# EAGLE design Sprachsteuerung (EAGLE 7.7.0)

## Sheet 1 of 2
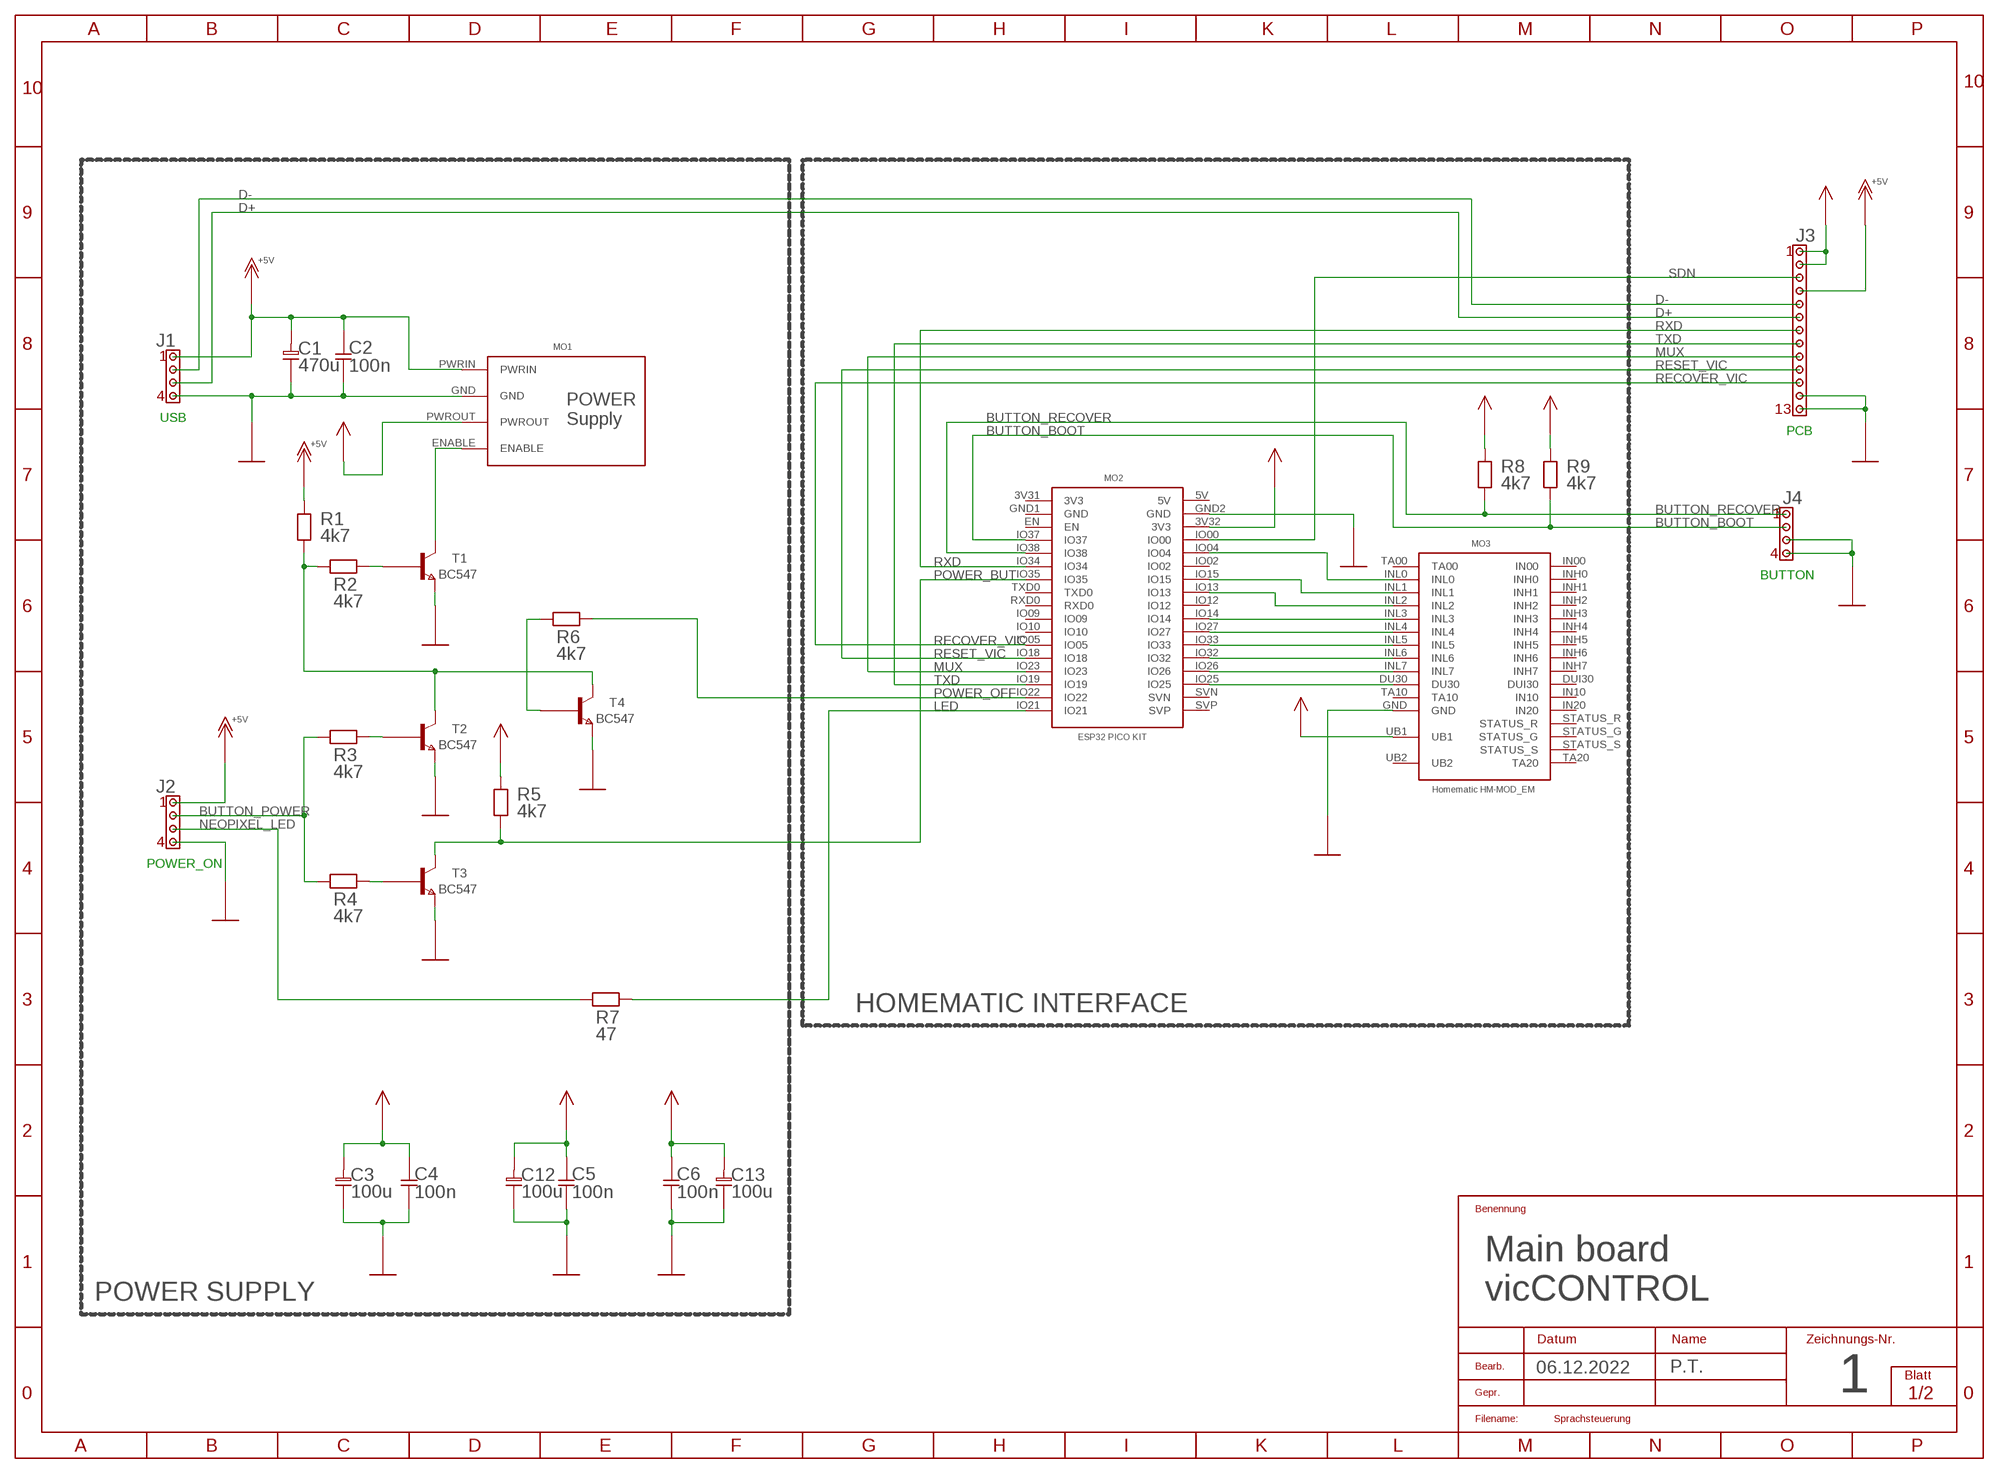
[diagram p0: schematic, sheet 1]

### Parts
C1  470u  ELK02ST  [ELKOS02B]
C2  100n  CAP02  [CAP02B]
C3  100u  ELK02ST  [ELKOS02B]
C4  100n  CAP02  [CAP02B]
C5  100n  CAP02  [CAP02B]
C6  100n  CAP02  [CAP02B]
C12  100u  ELK02ST  [ELKOS02B]
C13  100u  ELK02ST  [ELKOS02B]
J1  POWER_ON  CON04X1  [CON04X1]
J2  POWER_ON  CON04X1  [CON04X1]
J3  PCB  CON13X1  [CON13X1]
J4  BUTTON  CON04X1  [CON04X1]
MO1  POWER_SUPPLY  [POWER_SUPPLY]
MO2  ESP32-PICO-KIT  [ESP32-PICO-KIT]
MO3  HM_MOD_EM  [HM_MOD_EM]
R1  4k7  RES01  [RES01B]
R2  4k7  RES01  [RES01B]
R3  4k7  RES01  [RES01B]
R4  4k7  RES04  [RES04B]
R5  4k7  RES02  [RES02B]
R6  4k7  RES04  [RES04B]
R7  47  RES04  [RES04B]
R8  4k7  RES02  [RES02B]
R9  4k7  RES04  [RES04B]
T1  BC547  [TO92A]
T2  BC547  [TO92A]
T3  BC547  [TO92A]
T4  BC547  [TO92A]

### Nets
+5V: C1.P C2.2 J1.1 J2.1 J3.4 MO1.PWRIN R1.2
BUTTON_BOOT: J4.2 MO2.IO37 R9.1
BUTTON_POWER: J2.2 R3.1 R4.1
BUTTON_RECOVER: J4.1 MO2.IO38 R8.1
D+: J1.3 J3.6
D-: J1.2 J3.5
GND: C1.N C2.1 C3.N C4.1 C5.1 C6.1 C12.N C13.N J1.4 J2.4 J3.12 J3.13 J4.3 J4.4 MO1.GND MO2.GND2(GND) MO3.GND T1.3(E) T2.3(E) T3.3(E) T4.3(E)
LED: MO2.IO21 R7.2
MUX: J3.9 MO2.IO23
N$1: MO1.ENABLE T1.1(C)
N$2: R2.2 T1.2(B)
N$3: MO2.IO14 MO3.INL3
N$4: R1.1 R2.1 T2.1(C) T4.1(C)
N$5: MO2.IO04 MO3.INL0
N$10: R3.2 T2.2(B)
N$19: R4.2 T3.2(B)
N$21: MO2.IO15 MO3.INL1
N$22: R6.1 T4.2(B)
N$23: MO2.IO13 MO3.INL2
N$25: MO2.IO27 MO3.INL4
N$26: MO2.IO33 MO3.INL5
N$27: MO2.IO32 MO3.INL6
N$28: MO2.IO26 MO3.INL7
N$29: MO2.IO25 MO3.DU30
NEOPIXEL_LED: J2.3 R7.1
POWER_BUT: MO2.IO35 R5.1 T3.1(C)
POWER_OFF: MO2.IO22 R6.2
RECOVER_VIC: J3.11 MO2.IO05
RESET_VIC: J3.10 MO2.IO18
RXD: J3.7 MO2.IO34
SDN: J3.3 MO2.IO00
TXD: J3.8 MO2.IO19
VCC: C3.P C4.2 C5.2 C6.2 C12.P C13.P J3.1 J3.2 MO1.PWROUT MO2.3V32(3V3) MO3.UB1 R5.2 R8.2 R9.2
Unconnected: MO2.EN MO2.IO02 MO2.IO09 MO2.IO10 MO2.IO12 MO2.RXD0 MO2.SVN MO2.SVP MO2.TXD0 MO3.DUI30 MO3.IN00 MO3.IN10 MO3.IN20 MO3.INH0 MO3.INH1 MO3.INH2 MO3.INH3 MO3.INH4 MO3.INH5 MO3.INH6 MO3.INH7 MO3.STATUS_G MO3.STATUS_R MO3.STATUS_S MO3.TA00 MO3.TA10 MO3.TA20

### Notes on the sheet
- USB
- PCB
- BUTTON
- POWER_ON
- HOMEMATIC INTERFACE
- Main board
- POWER SUPPLY | vicCONTROL
- 06.12.2022 | P.T.
- 1

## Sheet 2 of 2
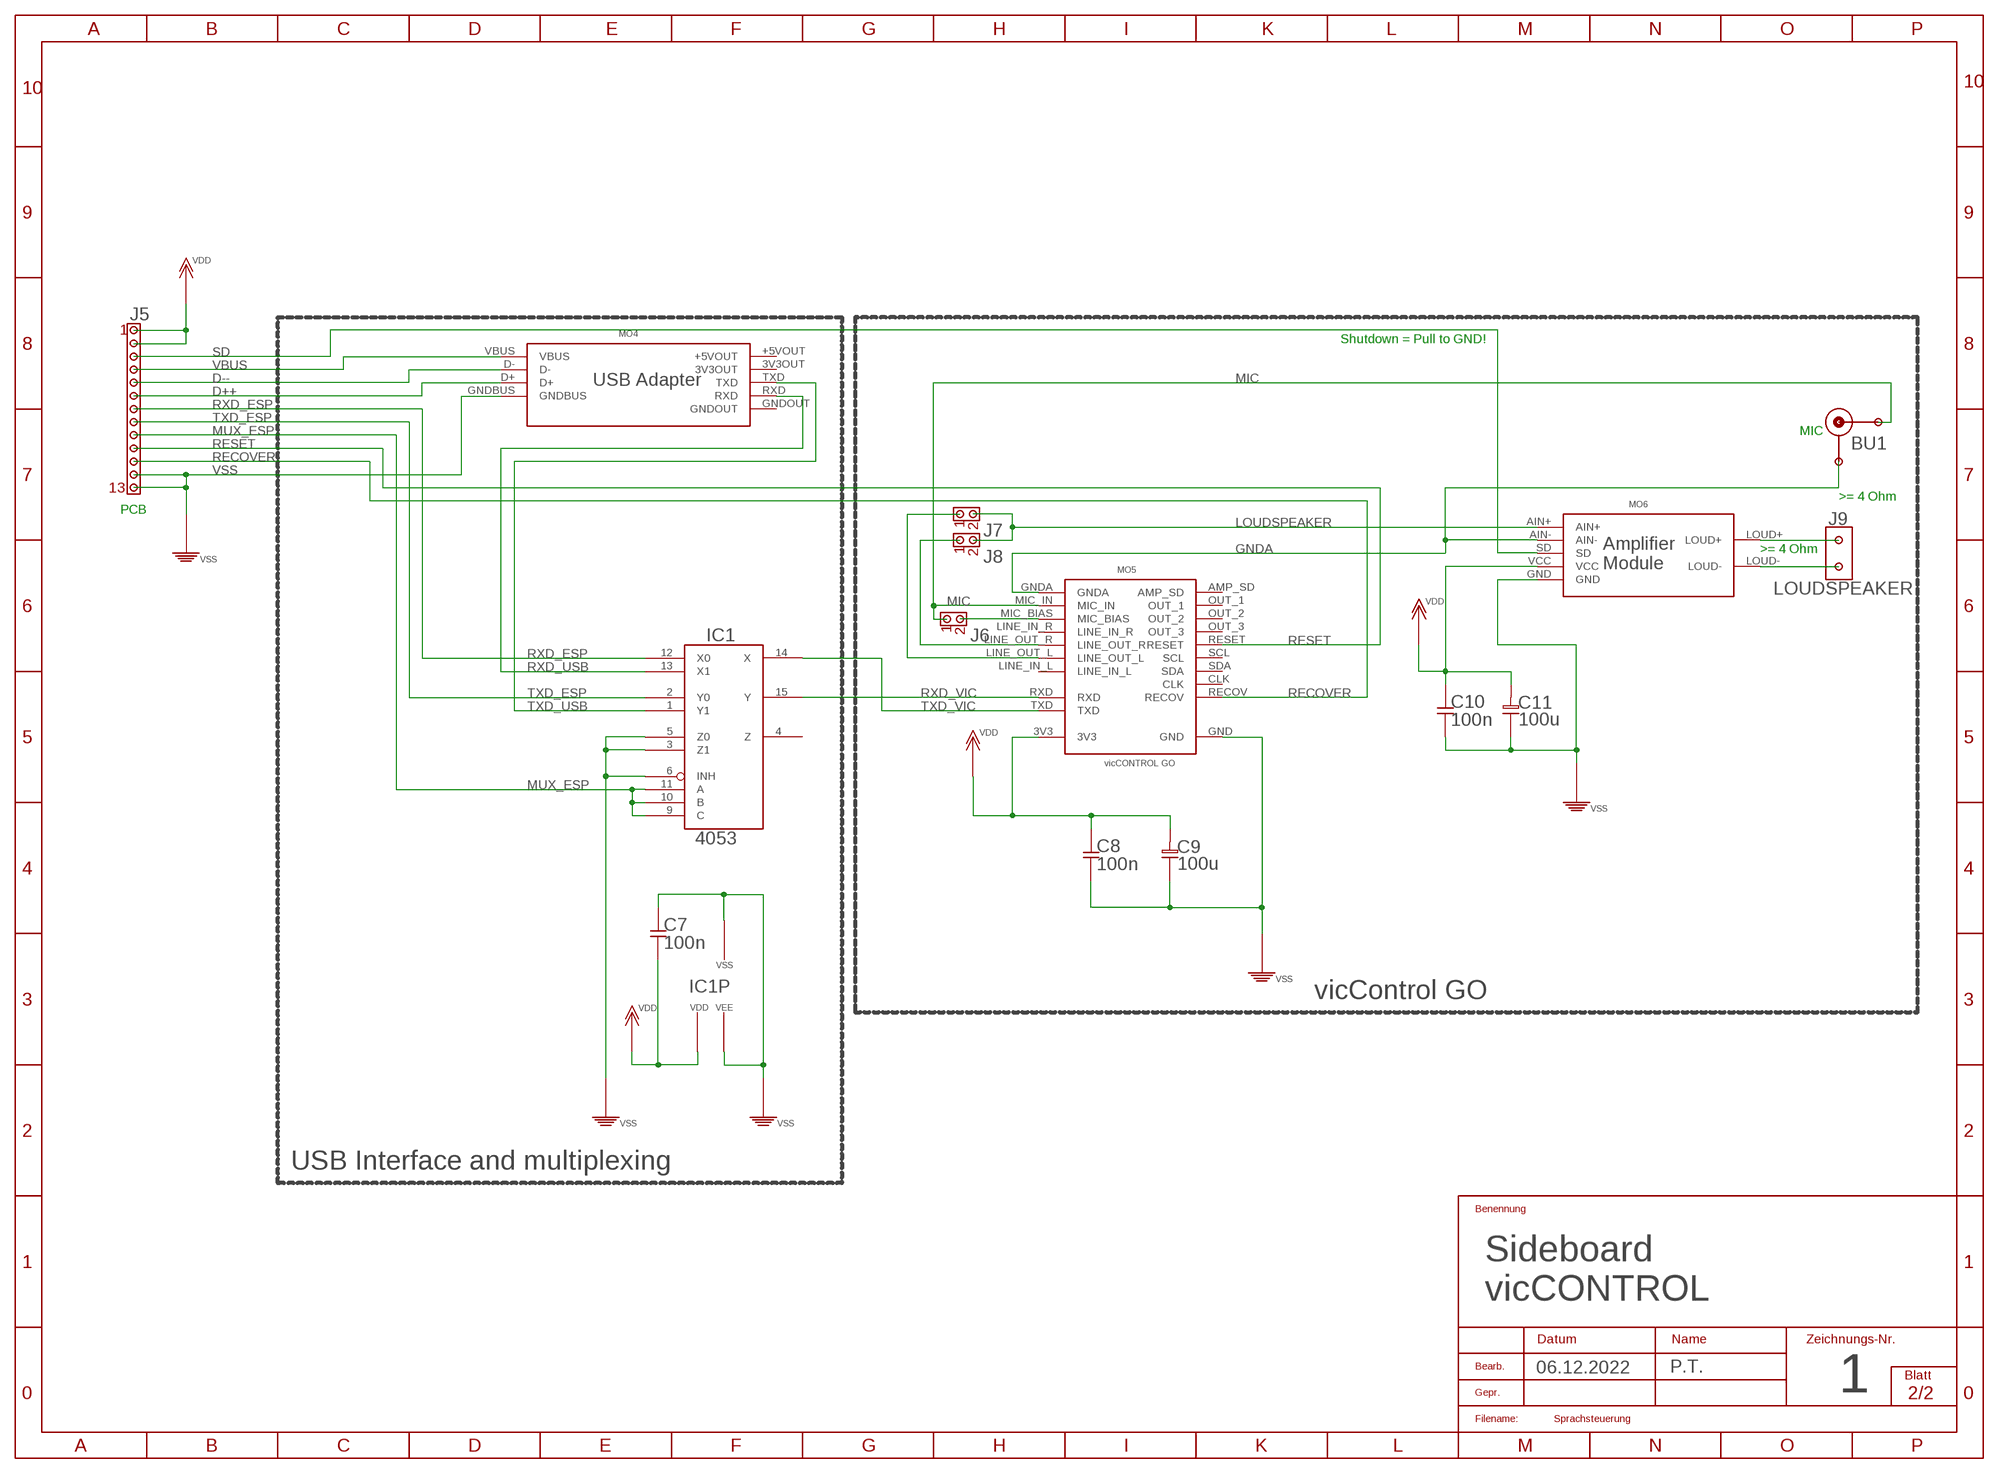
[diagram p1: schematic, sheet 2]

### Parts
BU1  MIC  KLINKE3M  [KLINKE3M]
C7  100n  CAP02  [CAP02B]
C8  100n  CAP02  [CAP02B]
C9  100u  ELK02ST  [ELKOS02B]
C10  100n  CAP02  [CAP02B]
C11  100u  ELK02ST  [ELKOS02B]
IC1  4053  [DIL16]
J5  PCB  CON13X1  [CON13X1]
J6  MIC  CON02X1  [CON02X1]
J7  LINE_L  CON02X1  [CON02X1]
J8  LINE_R  CON02X1  [CON02X1]
J9  LOUDSPEAKER  POWER2X1  [POWER2X1]
MO4  USB-ADAPTER  [USB-ADAPTER]
MO5  VIC-CONTROL-GO  [VIC-CONTROL-GO]
MO6  AMPLIFIER  [AMPLIFIER]

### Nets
D++: J5.6 MO4.D+
D--: J5.5 MO4.D-
GNDA: BU1.GND MO5.GNDA MO6.AIN-
LOUDSPEAKER: J7.2 J8.2 MO6.AIN+
MIC: BU1.IN J6.1 MO5.MIC_IN
MUX_ESP: IC1.9(C) IC1.10(B) IC1.11(A) J5.9
N$6: J6.2 MO5.MIC_BIAS
N$7: J8.1 MO5.LINE_OUT_R
N$8: J7.1 MO5.LINE_OUT_L
N$12: J9.2 MO6.LOUD+
N$13: J9.1 MO6.LOUD-
RECOVER: J5.11 MO5.RECOV
RESET: J5.10 MO5.RESET
RXD_ESP: IC1.12(X0) J5.7
RXD_USB: IC1.13(X1) MO4.RXD
RXD_VIC: IC1.15(Y) MO5.RXD
SD: J5.3 MO6.SD
TXD_ESP: IC1.2(Y0) J5.8
TXD_USB: IC1.1(Y1) MO4.TXD
TXD_VIC: IC1.14(X) MO5.TXD
VBUS: J5.4 MO4.VBUS
VDD: C7.1 C8.2 C9.P C10.2 C11.P IC1.16(VDD) J5.1 J5.2 MO5.3V3 MO6.VCC
VSS: C7.2 C8.1 C9.N C10.1 C11.N IC1.3(Z1) IC1.5(Z0) IC1.6(INH) IC1.7(VEE) IC1.8(VSS) J5.12 J5.13 MO4.GNDBUS MO5.GND MO6.GND
Unconnected: IC1.4(Z) MO5.AMP_SD MO5.CLK MO5.LINE_IN_L MO5.LINE_IN_R MO5.OUT_1 MO5.OUT_2 MO5.OUT_3 MO5.SCL MO5.SDA

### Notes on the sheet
- Shutdown = Pull to GND!
- MIC
- >= 4 Ohm
- PCB
- >= 4 Ohm
- vicControl GO
- USB Interface and multiplexing
- Sideboard
- vicCONTROL
- 06.12.2022 | P.T.
- 1

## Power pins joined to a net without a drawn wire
3V3: MO2.3V31(3V3)
3V3OUT: MO4.3V3OUT
5V: MO2.5V
+5VOUT: MO4.+5VOUT
GND: MO2.GND1(GND)
GNDOUT: MO4.GNDOUT
UB2: MO3.UB2

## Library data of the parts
BU1 = Mechanic:KLINKE3M
C1 C3 C9 C11-C13 = Discrete:ELK02ST
C2 C4-C8 C10 = Discrete:CAP02
IC1 = 40XX:4053
J1 J2 J4 = Connector 1:CON04X1
J3 J5 = Connector 1:CON13X1
J6-J8 = Connector 1:CON02X1
J9 = Connector 2:POWER2X1
MO1 = Giess:POWER_SUPPLY
MO2 = Giess:ESP32-PICO-KIT
MO3 = Giess:HM_MOD_EM
MO4 = Giess:USB-ADAPTER
MO5 = Giess:VIC-CONTROL-GO
MO6 = Giess:AMPLIFIER
R1-R3 = Discrete:RES01
R4 R6 R7 R9 = Discrete:RES04
R5 R8 = Discrete:RES02
T1-T4 = Transistor:BC547

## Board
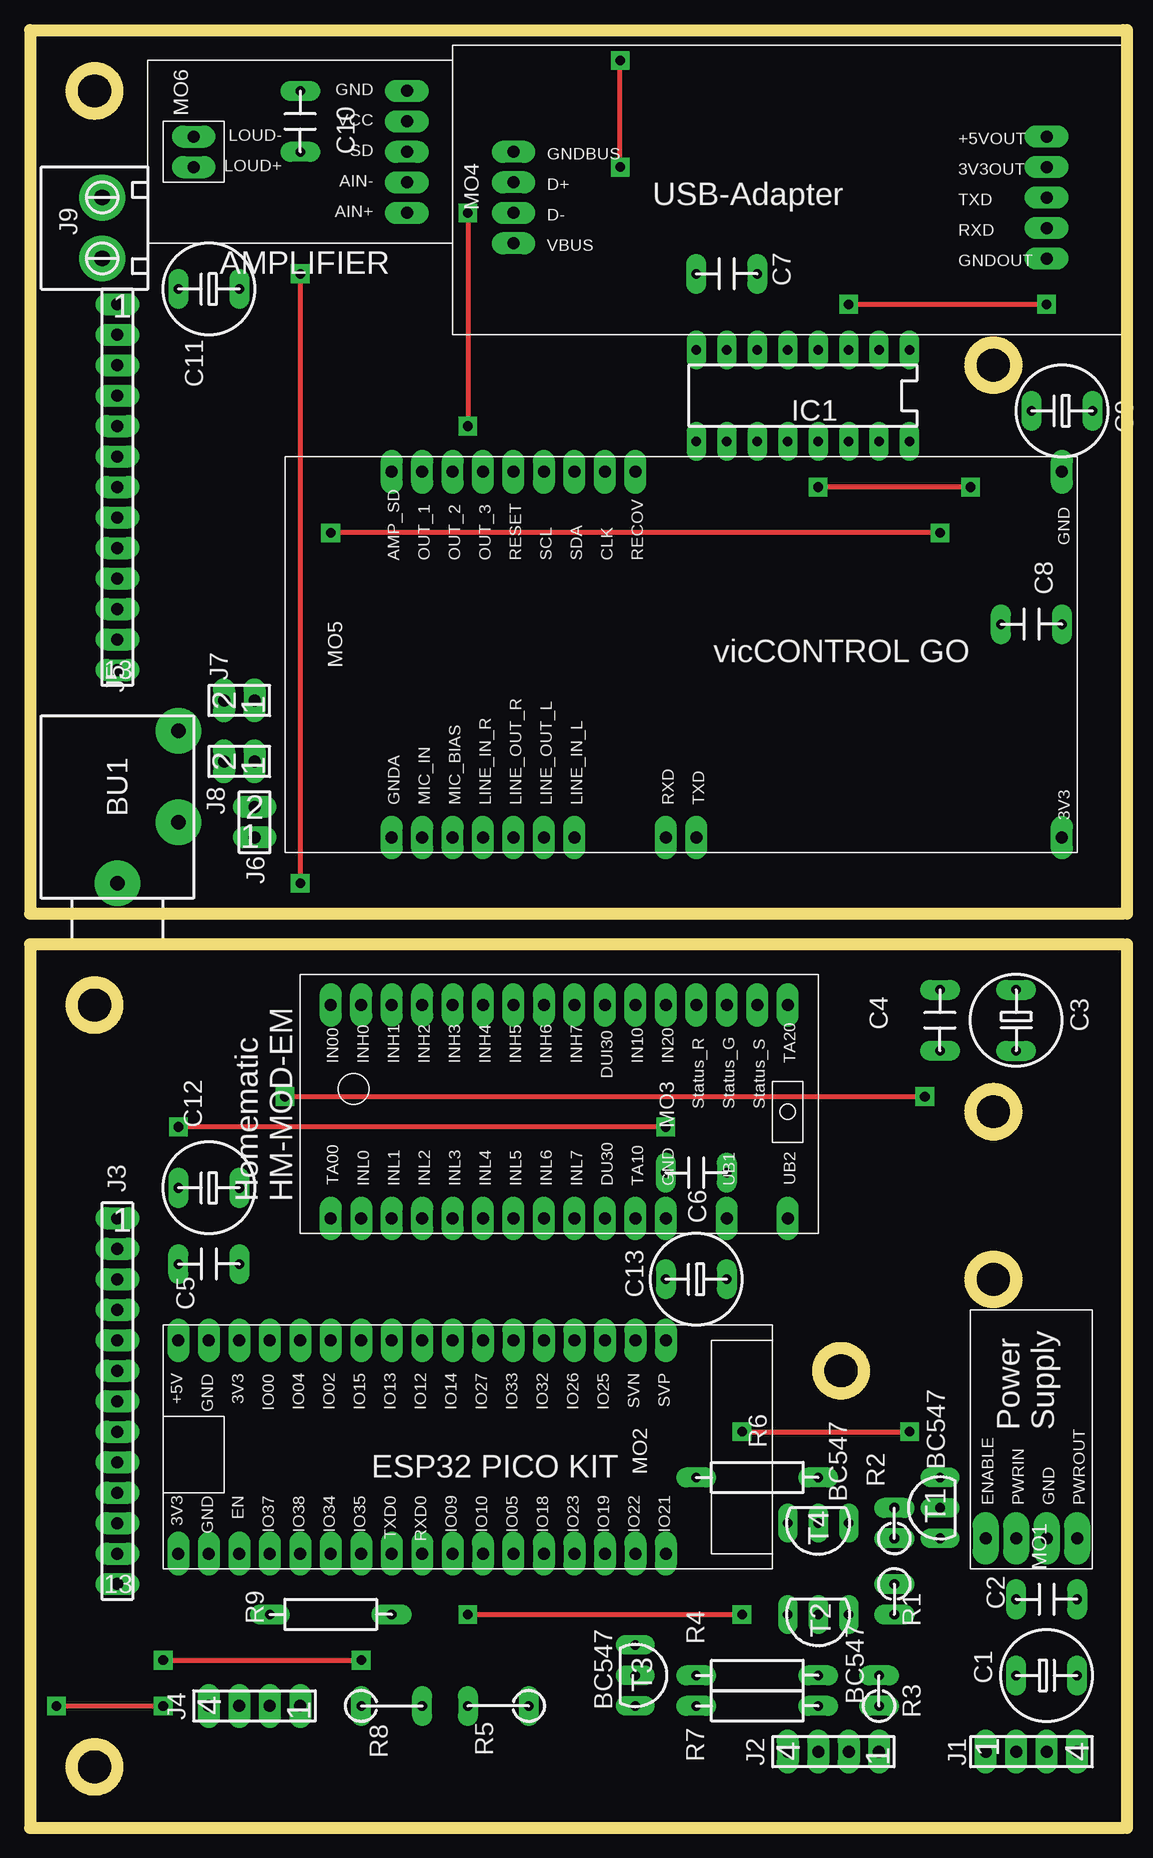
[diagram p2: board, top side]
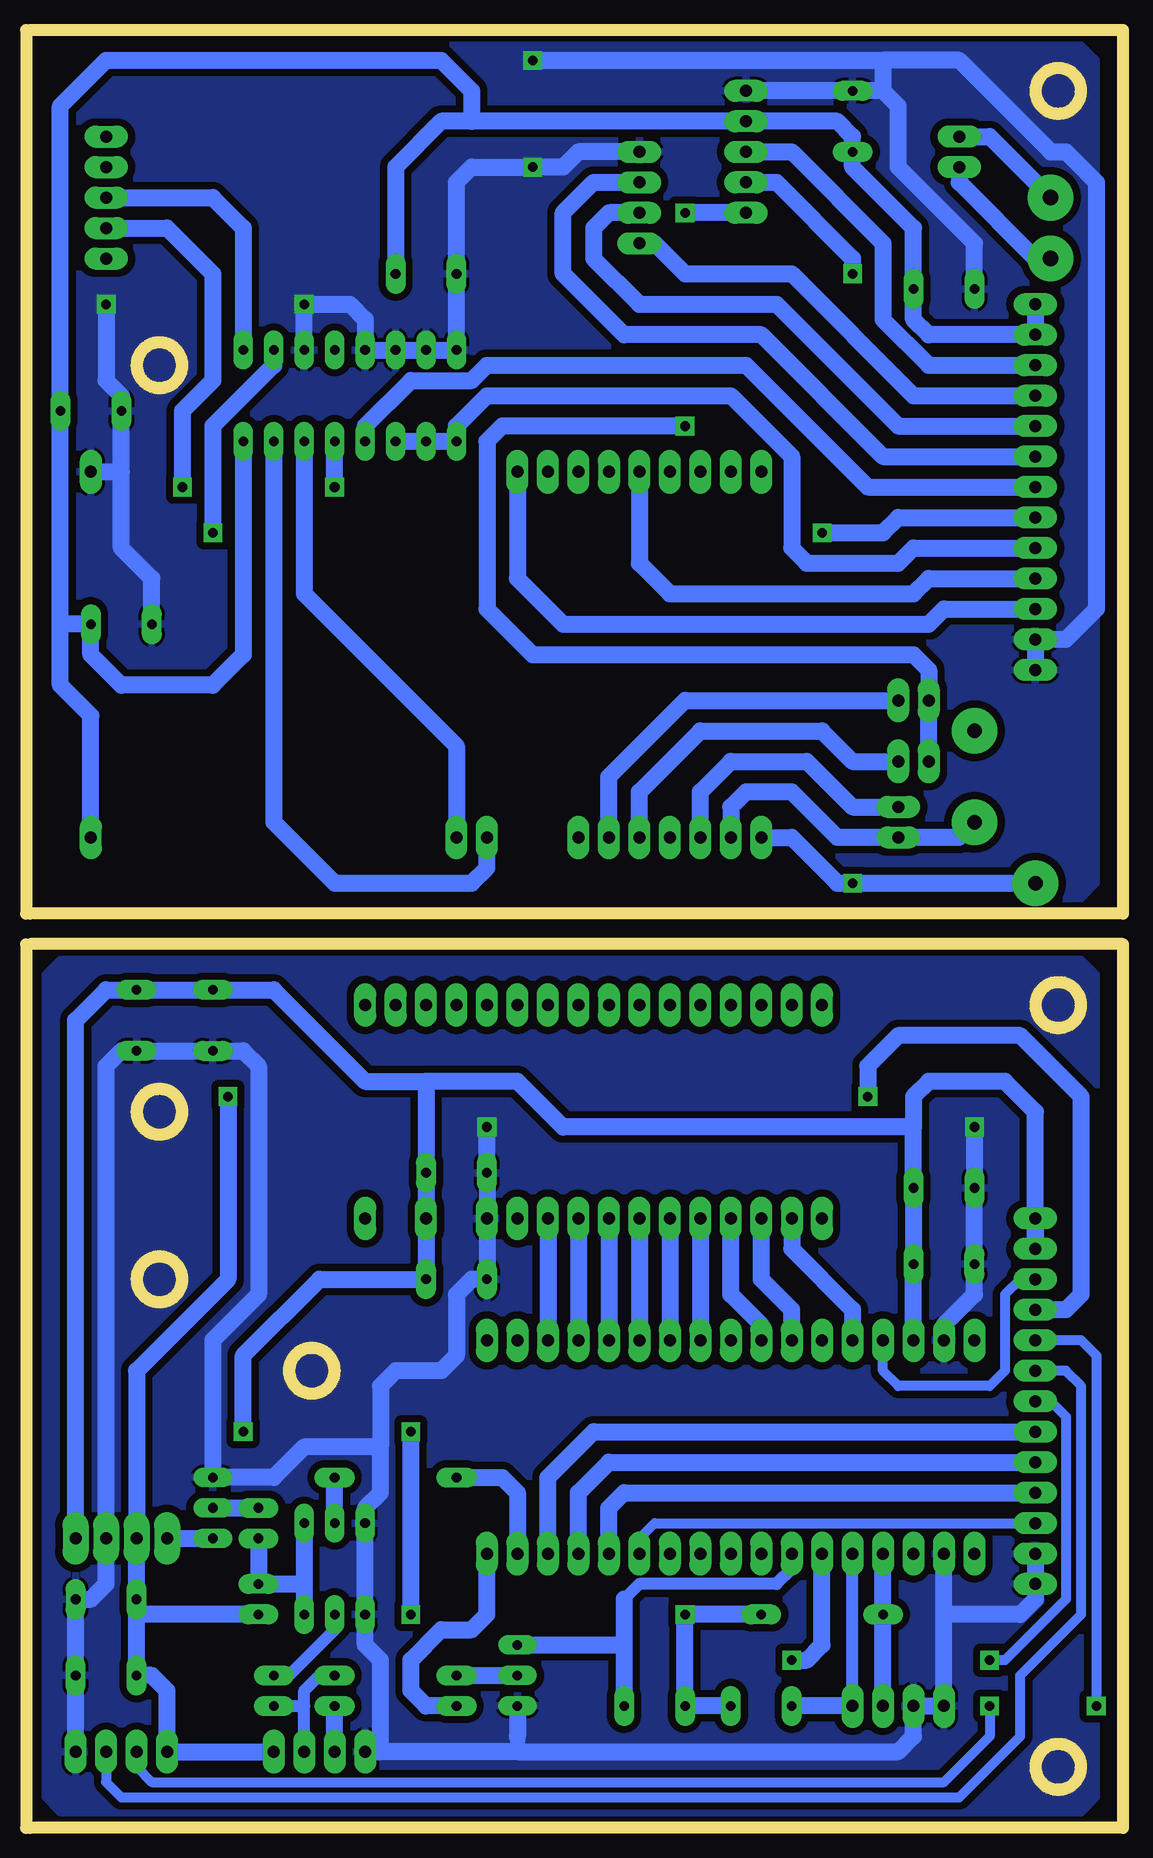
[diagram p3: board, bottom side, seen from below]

Size 91.11 x 149.86 mm. Coordinates in mm from the lower left corner, seen from the top.
Outline: 0,149.84 0,76.2
Outline: 91.11,76.18 0,76.18
Outline: 91.11,76.2 91.11,149.84
Outline: 0,149.86 91.11,149.86
Outline: 91.11,0 91.11,73.64 0,73.64 0,0 91.11,0
Copper layers (1*16): Top 0.035mm / dielectric 1.5mm / Bottom 0.035mm
Design rules "LP_fraesen": minimum track width 16mil, minimum drill 23mil, track to track 8mil, track to pad 8mil, pad to pad 8mil, via to via 8mil, smd to smd 0mil, copper to edge 20mil, drill to drill 8mil, minimum pad ring 16mil, minimum via ring 15mil, stop-mask expansion 4mil, vias tented up to drill 0mil, thermal gap 10mil
Milling: 22 lines

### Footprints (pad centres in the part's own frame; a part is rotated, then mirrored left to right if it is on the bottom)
KLINKE3M = drill 1.2 pad 3.81: GND 0,0; IN 5.08,-5.08; NC 12.7,-5.08
ELKOS02B = drill 0.8 pad 1.676 long: N 5.08,0; P 0,0
CAP02B = drill 0.8 pad 1.676 long: 1 0,0; 2 5.08,0
DIL16 = drill 0.8 pad 1.422 long: 1 0,0; 2 2.54,0; 3 5.08,0; 4 7.62,0; 5 10.16,0; 6 12.7,0; 7 15.24,0; 8 17.78,0; 9 17.78,7.62; 10 15.24,7.62; 11 12.7,7.62; 12 10.16,7.62; 13 7.62,7.62; 14 5.08,7.62; 15 2.54,7.62; 16 0,7.62
CON04X1 = drill 1 pad 1.422 long: 1 0,0; 2 0,-2.54; 3 0,-5.08; 4 0,-7.62
CON13X1 = drill 1 pad 1.422 long: 1 0,0; 2 0,-2.54; 3 0,-5.08; 4 0,-7.62; 5 0,-10.16; 6 0,-12.7; 7 0,-15.24; 8 0,-17.78; 9 0,-20.32; 10 0,-22.86; 11 0,-25.4; 12 0,-27.94; 13 0,-30.48
CON02X1 = drill 1 pad 1.422 long: 1 0,0; 2 0,-2.54
POWER2X1 = drill 1.3 pad 3.81: 1 0,0; 2 0,5.08
POWER_SUPPLY = drill 1 pad 2.184 long: ENABLE 0,0; GND 0,-5.08; PWRIN 0,-2.54; PWROUT 0,-7.62
ESP32-PICO-KIT = drill 1 pad 1.422 long: 3V31 22.86,5.08; 3V32 17.78,-12.7; 5V 22.86,-12.7; EN 17.78,5.08; GND1 20.32,5.08; GND2 20.32,-12.7; IO00 15.24,-12.7; IO02 10.16,-12.7; IO04 12.7,-12.7; IO05 -5.08,5.08; IO09 0,5.08; IO10 -2.54,5.08; IO12 2.54,-12.7; IO13 5.08,-12.7; IO14 0,-12.7; IO15 7.62,-12.7; IO18 -7.62,5.08; IO19 -12.7,5.08; IO21 -17.78,5.08; IO22 -15.24,5.08; IO23 -10.16,5.08; IO25 -12.7,-12.7; IO26 -10.16,-12.7; IO27 -2.54,-12.7; IO32 -7.62,-12.7; IO33 -5.08,-12.7; IO34 10.16,5.08; IO35 7.62,5.08; IO37 15.24,5.08; IO38 12.7,5.08; RXD0 2.54,5.08; SVN -15.24,-12.7; SVP -17.78,-12.7; TXD0 5.08,5.08
HM_MOD_EM = drill 1 pad 1.422 long: DU30 22.86,0; DUI30 22.86,17.78; GND 27.94,0; IN00 0,17.78; IN10 25.4,17.78; IN20 27.94,17.78; INH0 2.54,17.78; INH1 5.08,17.78; INH2 7.62,17.78; INH3 10.16,17.78; INH4 12.7,17.78; INH5 15.24,17.78; INH6 17.78,17.78; INH7 20.32,17.78; INL0 2.54,0; INL1 5.08,0; INL2 7.62,0; INL3 10.16,0; INL4 12.7,0; INL5 15.24,0; INL6 17.78,0; INL7 20.32,0; STATUS_G 33.02,17.78; STATUS_R 30.48,17.78; STATUS_S 35.56,17.78; TA00 0,0; TA10 25.4,0; TA20 38.1,17.78; UB1 33.02,0; UB2 38.1,0
USB-ADAPTER = drill 1 pad 1.422 long: 3V3OUT 24.13,1.27; +5VOUT 24.13,3.81; D+ -20.32,0; D- -20.32,-2.54; GNDBUS -20.32,2.54; GNDOUT 24.13,-6.35; RXD 24.13,-3.81; TXD 24.13,-1.27; VBUS -20.32,-5.08
VIC-CONTROL-GO = drill 1 pad 1.422 long: 3V3 38.1,-12.7; AMP_SD -17.78,17.78; CLK 0,17.78; GND 38.1,17.78; GNDA -17.78,-12.7; LINE_IN_L -2.54,-12.7; LINE_IN_R -10.16,-12.7; LINE_OUT_L -5.08,-12.7; LINE_OUT_R -7.62,-12.7; MIC_BIAS -12.7,-12.7; MIC_IN -15.24,-12.7; OUT_1 -15.24,17.78; OUT_2 -12.7,17.78; OUT_3 -10.16,17.78; RECOV 2.54,17.78; RESET -7.62,17.78; RXD 5.08,-12.7; SCL -5.08,17.78; SDA -2.54,17.78; TXD 7.62,-12.7
AMPLIFIER = drill 1 pad 1.422 long: AIN+ -20.32,2.54; AIN- -20.32,0; GND -20.32,-7.62; LOUD+ -2.54,-1.27; LOUD- -2.54,-3.81; SD -20.32,-2.54; VCC -20.32,-5.08
RES01B = drill 0.8 pad 1.676 long: 1 0,0; 2 2.54,0
RES04B = drill 0.8 pad 1.676 long: 1 0,0; 2 10.16,0
RES02B = drill 0.8 pad 1.676 long: 1 0,0; 2 5.08,0
TO92A = drill 0.8 pad 1.422 long: 1 0,0; 2 2.54,0; 3 5.08,0

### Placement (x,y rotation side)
BU1  7.29,78.74 90 top
C1  82.22,12.7 0 top
C2  87.3,19.05 180 top
C3  82.22,69.85 270 top
C4  75.87,64.77 90 top
C5  12.37,46.99 0 top
C6  53.01,54.61 0 top
C7  60.63,129.54 180 top
C8  80.95,100.33 0 top
C9  88.57,118.11 180 top
C10  22.53,144.78 270 top
C11  17.45,128.27 180 top
C12  17.45,53.34 180 top
C13  58.09,45.72 180 top
IC1  73.33,123.19 180 top
J1  79.68,6.35 90 top
J2  70.79,6.35 270 top
J3  7.29,50.8 0 top
J4  22.53,10.16 270 top
J5  7.29,127 0 top
J6  18.72,82.55 180 top
J7  18.72,93.98 270 top
J8  18.72,88.9 270 top
J9  6.02,135.89 180 top
MO1  79.68,24.13 90 top
MO2  35.23,27.94 180 top
MO3  25.07,50.8 0 top
MO4  60.63,137.16 0 top
MO5  47.93,95.25 0 top
MO6  11.1,137.16 180 top
R1  72.06,20.32 270 top
R2  72.06,24.13 90 top
R3  70.79,10.16 90 top
R4  65.71,12.7 180 top
R5  41.58,10.16 180 top
R6  65.71,29.21 180 top
R7  65.71,10.16 180 top
R8  27.61,10.16 0 top
R9  19.99,17.78 0 top
T1  75.87,24.13 90 top
T2  68.25,17.78 180 top
T3  50.47,15.24 270 top
T4  68.25,25.4 180 top

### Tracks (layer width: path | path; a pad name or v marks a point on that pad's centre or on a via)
+5V  (via drill 0.8 pad 1.42)
  Top 0.406: v21.26,60.96 v74.6,60.96
  Bottom 1.422: 82.22,17.78 C1.P 80.95,12.7 79.68,11.43 J1.1 J2.1 | 82.22,17.78 C2.2 MO1.PWRIN 82.22,38.1 74.6,45.72 v74.6,60.96 | R1.2 82.22,17.78 | v21.26,60.96 21.26,63.5 18.72,66.04 8.56,66.04 3.48,60.96 3.48,44.45 4.75,43.18 J3.4
BUTTON_BOOT
  Bottom 1.422: J4.2 R9.1 MO2.IO37
BUTTON_POWER
  Bottom 1.016: J2.2 68.25,10.16 | R3.1 68.25,10.16 | 68.25,10.16 68.25,11.43 66.98,12.7 R4.1
BUTTON_RECOVER
  Bottom 1.016: J4.1 MO2.IO38
  Bottom 1.422: J4.1 R8.1
D+
  Bottom 0.813: J1.3 84.76,3.81 83.49,2.54 13.64,2.54 8.56,7.62 8.56,12.7 3.48,17.78 3.48,36.83 4.75,38.1 J3.6
D++
  Bottom 1.422: MO4.D+ 44.12,137.16 46.66,134.62 46.66,129.54 41.58,124.46 30.15,124.46 19.99,114.3 J5.6
D-  (via drill 0.8 pad 1.42)
  Top 0.406: v2.21,10.16 v11.1,10.16
  Bottom 0.813: J1.2 82.22,5.08 80.95,3.81 14.91,3.81 11.1,7.62 v11.1,10.16 | v2.21,10.16 2.21,39.37 3.48,40.64 J3.5
D--
  Bottom 1.422: MO4.D- 42.85,134.62 44.12,133.35 44.12,130.81 40.31,127 28.88,127 18.72,116.84 J5.5
GND  (via drill 0.8 pad 1.42)
  Top 0.406: v53.01,58.42 v12.37,58.42
  Bottom 1.27: T3.3 50.47,6.35
  Bottom 1.422: J1.4 C1.N C2.1 86.03,19.05 84.76,20.32 MO1.GND 84.76,63.5 83.49,64.77 C3.N C4.1 73.33,64.77 72.06,63.5 72.06,44.45 75.87,40.64 T1.3 70.79,29.21 68.25,31.75 61.9,31.75 | J2.4 61.9,6.35 | 61.9,6.35 61.9,13.97 63.17,15.24 T2.3 T4.3 63.17,26.67 61.9,27.94 61.9,31.75 | 61.9,6.35 50.47,6.35 18.72,6.35 17.45,7.62 J4.3 J4.4 14.91,17.78 | T3.3 50.47,7.62 | 14.91,17.78 MO2.GND1 | J3.12 7.29,19.05 8.56,17.78 14.91,17.78 | 61.9,31.75 61.9,36.83 60.63,38.1 56.82,38.1 55.55,39.37 55.55,44.45 54.28,45.72 C13.N MO3.GND C6.1 v53.01,58.42 | MO2.GND2 14.91,41.91 12.37,44.45 C5.1 C12.N v12.37,58.42
  pour Bottom (isolate 0.61): 3.48,1.27 88.57,1.27 89.84,2.54 89.84,71.12 88.57,72.39 3.48,72.39 2.21,71.12 2.21,2.54
GNDA  (via drill 0.8 pad 1.42)
  Top 0.406: v22.53,129.54 v22.53,78.74
  Bottom 1.422: MO5.GNDA 27.61,82.55 23.8,78.74 v22.53,78.74 BU1.GND | MO6.AIN- 28.88,137.16 22.53,130.81 v22.53,129.54
LED
  Bottom 1.422: R7.2 58.09,10.16 59.36,11.43 59.36,13.97 56.82,16.51 54.28,16.51 53.01,17.78 MO2.IO21
LOUDSPEAKER  (via drill 0.8 pad 1.42)
  Top 0.406: v36.5,134.62 v36.5,116.84
  Bottom 1.422: J8.2 J7.2 16.18,96.52 17.45,97.79 49.2,97.79 53.01,101.6 53.01,115.57 51.74,116.84 v36.5,116.84 | MO6.AIN+ v36.5,134.62
MIC
  Bottom 1.422: BU1.IN 13.64,82.55 J6.1 23.8,82.55 27.61,86.36 31.42,86.36 32.69,85.09 MO5.MIC_IN
MUX
  Bottom 1.422: MO2.IO23 45.39,27.94 42.85,30.48 J3.9
MUX_ESP
  Bottom 1.422: IC1.11 IC1.10 IC1.9 55.55,116.84 53.01,119.38 32.69,119.38 27.61,114.3 27.61,106.68 26.34,105.41 18.72,105.41 17.45,106.68 J5.9
N$1
  Bottom 1.422: MO1.ENABLE T1.1
N$2
  Bottom 1.422: T1.2 R2.2
N$3
  Bottom 1.422: MO3.INL3 MO2.IO14
N$4
  Bottom 1.422: R2.1 R1.1 68.25,20.32 | 68.25,20.32 T2.1 | T4.1 68.25,20.32
N$5
  Bottom 1.422: MO3.INL0 27.61,48.26 22.53,43.18 MO2.IO04
N$6
  Bottom 1.422: MO5.MIC_BIAS 35.23,86.36 32.69,88.9 26.34,88.9 22.53,85.09 J6.2
N$7
  Bottom 1.422: MO5.LINE_OUT_R 40.31,86.36 35.23,91.44 25.07,91.44 22.53,88.9 J8.1
N$8
  Bottom 1.422: MO5.LINE_OUT_L 42.85,87.63 36.5,93.98 J7.1
N$10
  Bottom 1.016: T2.2 65.71,16.51 69.52,12.7 R3.2
N$12
  Bottom 1.422: MO6.LOUD+ 13.64,137.16 7.29,130.81 J9.2
N$13
  Bottom 1.422: MO6.LOUD- 11.1,140.97 J9.1
N$19
  Bottom 1.422: R4.2 T3.2
N$21
  Bottom 1.422: MO2.IO15 27.61,43.18 30.15,45.72 MO3.INL1
N$22
  Bottom 1.422: T4.2 R6.1
N$23
  Bottom 1.422: MO2.IO13 30.15,41.91 32.69,44.45 MO3.INL2
N$25
  Bottom 1.422: MO3.INL4 MO2.IO27
N$26
  Bottom 1.422: MO3.INL5 MO2.IO33
N$27
  Bottom 1.422: MO3.INL6 MO2.IO32
N$28
  Bottom 1.422: MO3.INL7 MO2.IO26
N$29
  Bottom 1.422: MO3.DU30 MO2.IO25
NEOPIXEL_LED
  Bottom 1.422: J2.3 R7.1
POWER_BUT
  Bottom 1.016: MO2.IO35 27.61,21.59 28.88,20.32 40.31,20.32 41.58,19.05
  Bottom 1.422: T3.1 41.58,15.24 | 41.58,15.24 R5.1 | 41.58,19.05 41.58,15.24
POWER_OFF
  Bottom 1.422: R6.2 51.74,29.21 50.47,27.94 MO2.IO22
RECOVER
  Bottom 1.422: MO5.RECOV 50.47,104.14 46.66,100.33 16.18,100.33 14.91,101.6 J5.11
RECOVER_VIC
  Bottom 0.813: MO2.IO05 40.31,24.13 39.04,25.4 J3.11
RESET
  Bottom 1.422: MO5.RESET 40.31,105.41 37.77,102.87 17.45,102.87 16.18,104.14 J5.10
RESET_VIC
  Bottom 1.422: MO2.IO18 42.85,26.67 41.58,27.94 J3.10
RXD  (via drill 0.8 pad 1.42)
  Top 0.406: v11.1,13.97 v27.61,13.97
  Bottom 0.813: v11.1,13.97 9.83,13.97 4.75,19.05 4.75,34.29 6.02,35.56 J3.7
  Bottom 1.422: v27.61,13.97 26.34,13.97 25.07,15.24 MO2.IO34
RXD_ESP
  Bottom 1.422: IC1.12 63.17,116.84 59.36,120.65 54.28,120.65 53.01,121.92 31.42,121.92 21.26,111.76 J5.7
RXD_USB  (via drill 0.8 pad 1.42)
  Top 0.406: v78.41,111.76 v65.71,111.76
  Bottom 1.422: MO4.RXD 79.68,133.35 75.87,129.54 75.87,120.65 78.41,118.11 v78.41,111.76 | v65.71,111.76 IC1.13
RXD_VIC
  Bottom 1.422: IC1.15 70.79,83.82 65.71,78.74 54.28,78.74 53.01,80.01 MO5.RXD
SD
  Bottom 1.422: MO6.SD 27.61,139.7 19.99,132.08 19.99,125.73 16.18,121.92 J5.3
SDN
  Bottom 0.813: J3.3 8.56,45.72 9.83,44.45 9.83,38.1 11.1,36.83 18.72,36.83 19.99,38.1 MO2.IO00
TXD
  Bottom 1.422: MO2.IO19 47.93,29.21 44.12,33.02 J3.8
TXD_ESP  (via drill 0.8 pad 1.42)
  Top 0.406: v75.87,107.95 v25.07,107.95
  Bottom 1.422: IC1.2 70.79,121.92 75.87,116.84 v75.87,107.95 | v25.07,107.95 19.99,107.95 18.72,109.22 J5.8
TXD_USB
  Bottom 1.422: MO4.TXD 75.87,135.89 73.33,133.35 IC1.1
TXD_VIC
  Bottom 1.422: IC1.14 68.25,102.87 55.55,90.17 MO5.TXD
VBUS
  Bottom 1.422: MO4.VBUS 39.04,132.08 36.5,129.54 27.61,129.54 17.45,119.38 J5.4
VCC  (via drill 0.8 pad 1.42)
  Top 0.406: v36.5,17.78 v59.36,17.78 | v59.36,33.02 v73.33,33.02
  Bottom 1.422: MO1.PWROUT 87.3,67.31 84.76,69.85 C3.P C4.2 70.79,69.85 63.17,62.23 58.09,62.23 | R8.2 R5.2 v36.5,17.78 R9.2 | 17.45,58.42 C12.P C5.2 MO2.3V32 | 17.45,58.42 17.45,60.96 16.18,62.23 9.83,62.23 7.29,59.69 J3.2 J3.1 | 17.45,58.42 46.66,58.42 50.47,62.23 58.09,62.23 | 58.09,62.23 C6.2 MO3.UB1 C13.P 66.98,45.72 73.33,39.37 v73.33,33.02 | v59.36,17.78 v59.36,33.02
VDD
  Bottom 1.422: MO5.3V3 86.03,92.71 88.57,95.25 88.57,100.33 | 88.57,100.33 C8.2 86.03,97.79 83.49,95.25 75.87,95.25 73.33,97.79 IC1.16 | 88.57,100.33 C9.P 88.57,143.51 84.76,147.32 56.82,147.32 54.28,144.78 54.28,142.24 | J5.1 J5.2 16.18,124.46 17.45,125.73 C11.P 17.45,133.35 22.53,138.43 C10.2 22.53,140.97 23.8,142.24 MO6.VCC 54.28,142.24 | 54.28,142.24 56.82,142.24 60.63,138.43 C7.1
VSS  (via drill 0.8 pad 1.42)
  Top 0.406: v49.2,138.43 v49.2,147.32 | v68.25,127 v84.76,127
  Bottom 1.422: C8.1 80.95,104.14 83.49,106.68 83.49,113.03 | MO5.GND 83.49,113.03 | 83.49,113.03 C9.N 83.49,119.38 84.76,120.65 v84.76,127 | C11.N 12.37,132.08 18.72,138.43 18.72,143.51 19.99,144.78 | 19.99,144.78 C10.1 MO6.GND | MO4.GNDBUS 45.39,139.7 46.66,138.43 v49.2,138.43 54.28,138.43 55.55,137.16 C7.2 IC1.8 IC1.7 IC1.6 IC1.5 63.17,125.73 64.44,127 v68.25,127 IC1.3 | v49.2,147.32 19.99,147.32 | 19.99,147.32 13.64,147.32 6.02,139.7 4.75,139.7 2.21,137.16 2.21,101.6 4.75,99.06 J5.12 J5.13 | 19.99,147.32 19.99,144.78
  pour Bottom (isolate 0.61): 2.21,78.74 2.21,147.32 3.48,148.59 88.57,148.59 89.84,147.32 89.84,80.01 88.57,77.47 3.48,77.47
